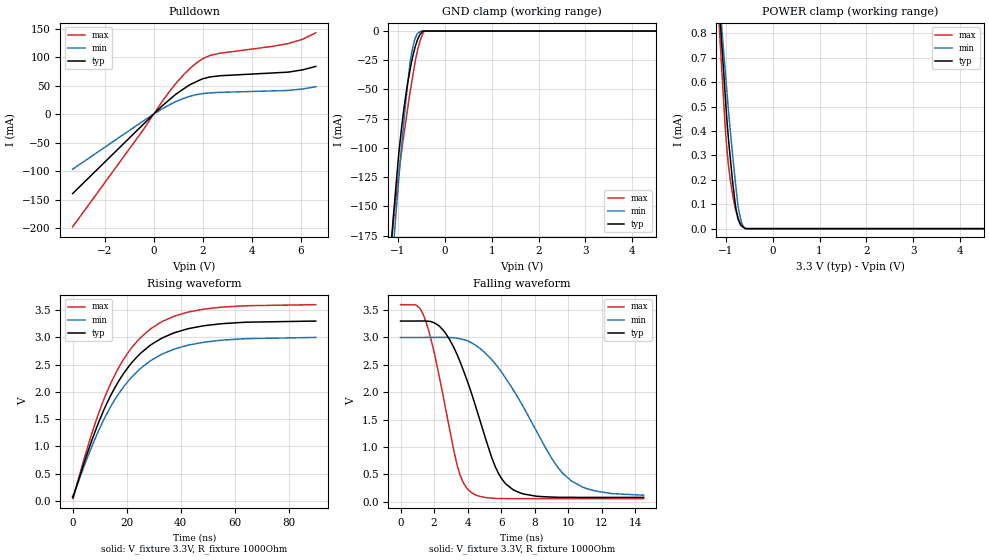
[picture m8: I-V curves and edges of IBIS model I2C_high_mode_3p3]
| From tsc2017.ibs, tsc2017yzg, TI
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|   i2c_high_mode_3p3 Model
[Model]   I2C_high_mode_3p3
Model_type   I/O_open_drain
Polarity   Non-Inverting
Enable   Active-Low
Vinl = 0.99
Vinh = 2.31
Vmeas = 1.65
Vref = 3.3
Cref = 100pF
Rref = 1000
|   typ   min   max
|   (nom PVT)   (Fast PVT)   (slow PVT)
|Average
C_comp   1.438e-11   1.385e-11   1.490e-11
|ON state : BUFFER OUTPUT TURNED LOW
|C_comp   3.212e-11   3.023e-11   3.426e-11
|OFF state: BUFFER in HIGH IMPEDANCE
|C_comp   1.438e-11   1.385e-11   1.490e-11
|C_comp from frequency method(F=3.4MHz)
| Where nom  PVT is Nominal Process, 3.3V, 25C
|   Fast PVT is Strong Process,  3.6V, -40C
|   Slow PVT is Weak Process,   3V, 85C
[Model Spec]
Vinl   0.99   0.9   1.08
Vinh   2.31   2.1   2.52
[Voltage Range]   3.3   3   3.6
|Ambient Temperature   25   85   -40
|Junction Temperature
[Temperature Range]   25   85   -40
[Pullup Reference]   3.3   3   3.6
[Pulldown Reference]   0   0   0
[Power Clamp Reference]   3.3   3   3.6
[GND Clamp Reference]   0   0   0
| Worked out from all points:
|   slope of the pulldown table from 0 to 0.495 V, typ, clamps not added: 24.9 ohm
|   GND clamp passes 1 mA (typ) near -0.49 V on its own axis
|   POWER clamp passes 1 mA (typ) near -1.17 V on its own axis
|   falling waveform, V_fixture 3.3V, R_fixture 1000Ohm: 20-80 % time 2.13ns typ, 3.34ns min, 1.43ns max; typ from 3.3 V to 0.077 V
|   rising waveform, V_fixture 3.3V, R_fixture 1000Ohm: 20-80 % time 19.7ns typ, 20.3ns min, 19ns max; typ from 0.075 V to 3.3 V
[Pulldown]
|   Voltage   I(typ)   I(min)   I(max)
-3.3V     -139.5mA   -96.81mA   -197.8mA
-384mV    -16.41mA   -10.95mA   -25.15mA
368.4mV   15.2mA     9.755mA    23.5mA
663.6mV   26.06mA    16.67mA    40.79mA
1.229V    44.44mA    27.71mA    69.46mA
1.74V     56.88mA    34.22mA    89.53mA
2.024V    62.18mA    36.03mA    97.81mA
2.291V    65.14mA    37.06mA    102.9mA
2.676V    67.11mA    38.07mA    106.6mA
5.477V    73.65mA    41.56mA    123.7mA
6.064V    77.56mA    44.05mA    131.3mA
6.6V      83.68mA    47.97mA    142.6mA
[GND Clamp]
|   Voltage   I(typ)   I(min)   I(max)
-3.3V     -1.445A    -1.41A     -1.544A
-1.151V   -187.2mA   -214.2mA   -187mA
-1.096V   -159.7mA   -185.5mA   -164.7mA
-1.072V   -148.3mA   -173.3mA   -155mA
-973.5mV  -103.1mA   -124.2mA   -120.3mA
-914.1mV  -81.15mA   -96.36mA   -101.8mA
-851.4mV  -61.21mA   -69.81mA   -83.74mA
-738mV    -33.27mA   -26.88mA   -52.42mA
-627mV    -13.21mA   -5.979mA   -25.77mA
-502.8mV  -1.724mA   0A         -5.94mA
-432mV    0A         0A         0A
6.6V      0A         0A         0A
[POWER Clamp]
|   Voltage   I(typ)   I(min)   I(max)
-3.3V     7.227mA    6.118mA    8.75mA
-1.137V   912.4uA    952.9uA    834.7uA
-1.115V   847.5uA    899uA      753.3uA
-1.018V   568.8uA    665.7uA    440.8uA
-999.6mV  517.2uA    623uA      386.7uA
-973.5mV  443.8uA    561.6uA    325.7uA
-906mV    298.3uA    410.6uA    205.8uA
-778.8mV  78.64uA    166uA      72.09uA
-738mV    41.46uA    94.85uA    45.43uA
-702mV    24.37uA    56.74uA    27.51uA
-594mV    1.669uA    0A         1.83uA
6.6V      0A         0A         0A
[Ramp]
R_load = 1000
|   typ   min   max
dV/dt_r   1.93315/1.96657e-08   1.7348/2.02922e-08   2.12634/1.89962e-08
dV/dt_f   1.9349/2.12281e-09   1.7368/3.34653e-09   2.1278/1.4206e-09
[Falling Waveform]
V_fixture = 3.3V
V_fixture_min = 3V
V_fixture_max = 3.6V
R_fixture = 1000Ohm
|   Time   V(typ)   V(min)   V(max)
0s        3.3V       3V         3.6V
1.425ns   3.301V     3.001V     3.364V
2.375ns   3.191V     3.002V     2.189V
3.4ns     2.669V     2.985V     639.5mV
4.25ns    1.963V     2.9V       160.4mV
5.65ns    638.8mV    2.518V     58.94mV
6.7ns     220.2mV    2.054V     53.48mV
9ns       82.85mV    799.2mV    54.45mV
10.2ns    77.95mV    375.5mV    54.4mV
14.5ns    77.27mV    116.7mV    53.94mV
[Rising Waveform]
V_fixture = 3.3V
V_fixture_min = 3V
V_fixture_max = 3.6V
R_fixture = 1000Ohm
|   Time   V(typ)   V(min)   V(max)
0s        75.16mV    105.3mV    53.66mV
200ps     65.97mV    104.2mV    39.48mV
425ps     102.4mV    105mV      97.37mV
8.05ns    1.235V     1.109V     1.377V
13.9ns    1.913V     1.71V      2.13V
20.58ns   2.452V     2.196V     2.721V
28.15ns   2.831V     2.545V     3.125V
36.8ns    3.066V     2.767V     3.37V
47.95ns   3.206V     2.903V     3.51V
89.97ns   3.297V     2.997V     3.598V
